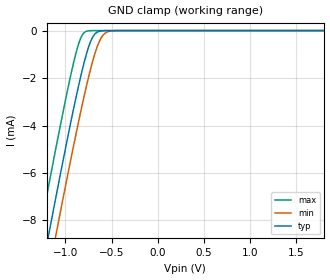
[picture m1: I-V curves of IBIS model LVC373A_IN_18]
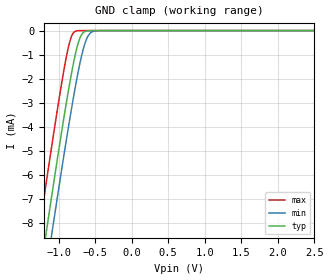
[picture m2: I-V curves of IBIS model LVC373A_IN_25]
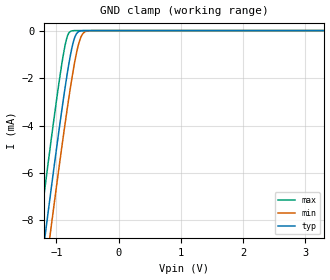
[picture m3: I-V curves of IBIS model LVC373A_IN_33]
| TEXAS INSTRUMENTS INCORPORATED
| Standard Linear and Logic Group
| IBIS Model of SN74LVC373A
| OCTAL TRANSPARENT D-TYPE LATCHES WITH 3-STATE OUTPUTS
| This file contains package information for the following:
|  TSSOP 20-pin (PW) package as [Component] LVC373A_PW
|  SSOP 20-pin (DB) package as [Component] LVC373A_DB
|  SOIC 20-pin (DW) package as [Component] LVC373A_DW
| This device can be powered at the following Vccs:
|  1.8 volt Vcc
|  2.5 volt Vcc
|  3.3 volt Vcc
| This file provides unique models under the [Model Selector] for each Vcc.
| For operation at a specific Vcc, select the appropriate model after each
| [Model Selector] keyword.
[IBIS Ver]   3.2
[Comment char]  |_char
[File Name]   sn74lvc373a.ibs
[File Rev]   1.1 | e-die
[Date]   March 5, 2002
[Source]   Data created from TI-SPICE simulations at TI-SLL.
[Notes]   The following is an IBIS list for the LVC373A.
   Please contact sllibis@ti.com with questions and
   comments concerning SLL IBIS models.
   -As there is no power clamp diode in the Input and I/O Models,
   we removed the Pwr Clamp table data from those Models.
   -Due to the fact that the Device is 5-V Input/Output
   tolarent, the output model has some Non-Monotonic Warnings.
   - C_comp values are taken at a different test condition than
   the data sheet.
[Disclaimer] Property of Texas Instruments Incorporated.  Unauthorized
   reproduction and/or distribution is strictly prohibited.
   This product is protected under copyright law.
   Created  2002, (C) Copyright  2002, Texas Instruments
   Incorporated, All Rights Reserved
   UNLESS THERE IS A SIGNED, WRITTEN AGREEMENT TO THE
   CONTRARY, TEXAS INSTRUMENTS (TI) IS PROVIDING THE IBIS
   MODELS  AND WITHOUT ANY WARRANTY, EXPRESSED OR
   IMPLIED.  TI assumes no liability for:
   1) the accuracy of the IBIS models provided to your
   company;
   2) the proper functioning of these IBIS Models in your
   design or for any resulting applications; or
   3) infringement of patents, copyrights or intellectual
   property rights resulting from your use of these IBIS
   models.
   TI provides IBIS Models as a service to our customers.
   You and your company shall not distribute, sell or give
   these models to anyone else without prior written
   permission from TI.
   TI reserves the right to make changes to our products or
   to discontinue any semiconductor product or service
   without notice, and advises our customers to obtain the
   latest version of relevant information to verify, before
   placing orders, that the information being relied on is
   current.
   Please be aware that your receipt and use of the IBIS
   information provided shall serve as acceptance of these
   terms and conditions.  If you do not accept these terms,
   you should return or destroy the IBIS models and any
   other accompanying information immediately.
| Component LVC373A_PW 20-pin TSSOP
[Component]   LVC373A_PW
[Manufacturer]   Texas Instruments, Inc.
[Package]
|   typ   min   max
R_pkg   4.500e-02   3.600e-02   5.700e-02
L_pkg   2.694e-09   2.290e-09   3.177e-09
C_pkg   1.560e-13   7.600e-14   2.590e-13
[Pin]   signal_name   model_name   R_pin   L_pin   C_pin
1   NOE   LVC373A_CTL   3.600e-02   3.045e-09   2.590e-13
2   1Q   LVC373A_OUT   5.100e-02   3.013e-09   1.890e-13
3   1D   LVC373A_IN   4.400e-02   2.695e-09   1.640e-13
4   2D   LVC373A_IN   4.700e-02   2.362e-09   7.900e-14
5   2Q   LVC373A_OUT   4.700e-02   2.333e-09   8.600e-14
6   3Q   LVC373A_OUT   4.700e-02   2.298e-09   8.500e-14
7   3D   LVC373A_IN   4.700e-02   2.351e-09   7.900e-14
8   4D   LVC373A_IN   4.400e-02   2.706e-09   1.650e-13
9   4Q   LVC373A_OUT   4.900e-02   2.999e-09   1.880e-13
10   GND   GND   3.900e-02   3.039e-09   2.570e-13
11   LE   LVC373A_CTL   3.800e-02   3.044e-09   2.580e-13
12   5Q   LVC373A_OUT   5.700e-02   3.177e-09   1.990e-13
13   5D   LVC373A_IN   4.400e-02   2.825e-09   1.730e-13
14   6D   LVC373A_IN   4.700e-02   2.429e-09   8.300e-14
15   6Q   LVC373A_OUT   4.900e-02   2.383e-09   9.000e-14
16   7Q   LVC373A_OUT   4.900e-02   2.347e-09   8.900e-14
17   7D   LVC373A_IN   4.700e-02   2.290e-09   7.600e-14
18   8D   LVC373A_IN   4.500e-02   2.613e-09   1.580e-13
19   8Q   LVC373A_OUT   4.400e-02   2.883e-09   1.810e-13
20   VCC   POWER   3.900e-02   3.044e-09   2.560e-13
| Component LVC373A_DB 20-pin SSOP
[Component]   LVC373A_DB
[Manufacturer]   Texas Instruments, Inc.
[Package]
|   typ   min   max
R_pkg   4.000e-02   3.500e-02   5.100e-02
L_pkg   3.495e-09   3.035e-09   4.314e-09
C_pkg   4.200e-13   3.460e-13   5.020e-13
[Pin]   signal_name   model_name   R_pin   L_pin   C_pin
1   NOE   LVC373A_CTL   4.900e-02   4.310e-09   5.020e-13
2   1Q   LVC373A_OUT   4.800e-02   3.903e-09   4.870e-13
3   1D   LVC373A_IN   3.500e-02   3.189e-09   3.960e-13
4   2D   LVC373A_IN   3.500e-02   3.036e-09   3.470e-13
5   2Q   LVC373A_OUT   3.500e-02   3.035e-09   3.670e-13
6   3Q   LVC373A_OUT   3.500e-02   3.035e-09   3.670e-13
7   3D   LVC373A_IN   3.500e-02   3.036e-09   3.470e-13
8   4D   LVC373A_IN   3.500e-02   3.189e-09   3.970e-13
9   4Q   LVC373A_OUT   4.700e-02   3.899e-09   4.880e-13
10   GND   GND   5.100e-02   4.314e-09   5.000e-13
11   LE   LVC373A_CTL   5.100e-02   4.314e-09   5.000e-13
12   5Q   LVC373A_OUT   4.700e-02   3.899e-09   4.880e-13
13   5D   LVC373A_IN   3.500e-02   3.189e-09   3.970e-13
14   6D   LVC373A_IN   3.500e-02   3.036e-09   3.460e-13
15   6Q   LVC373A_OUT   3.500e-02   3.035e-09   3.670e-13
16   7Q   LVC373A_OUT   3.500e-02   3.035e-09   3.670e-13
17   7D   LVC373A_IN   3.500e-02   3.036e-09   3.460e-13
18   8D   LVC373A_IN   3.500e-02   3.189e-09   3.970e-13
19   8Q   LVC373A_OUT   4.700e-02   3.899e-09   4.880e-13
20   VCC   POWER   5.100e-02   4.314e-09   5.020e-13
| Component LVC373A_DW 20-pin SOIC
[Component]   LVC373A_DW
[Manufacturer]   Texas Instruments, Inc.
[Package]
|   typ   min   max
R_pkg   3.800e-02   3.300e-02   4.500e-02
L_pkg   5.012e-09   4.110e-09   6.349e-09
C_pkg   7.170e-13   5.300e-13   8.680e-13
[Pin]   signal_name   model_name   R_pin   L_pin   C_pin
1   NOE   LVC373A_CTL   4.200e-02   6.336e-09   8.650e-13
2   1Q   LVC373A_OUT   4.300e-02   5.542e-09   8.670e-13
3   1D   LVC373A_IN   3.400e-02   4.714e-09   7.320e-13
4   2D   LVC373A_IN   3.400e-02   4.377e-09   5.910e-13
5   2Q   LVC373A_OUT   3.600e-02   4.130e-09   5.330e-13
6   3Q   LVC373A_OUT   3.500e-02   4.111e-09   5.300e-13
7   3D   LVC373A_IN   3.400e-02   4.284e-09   5.830e-13
8   4D   LVC373A_IN   3.400e-02   4.634e-09   7.260e-13
9   4Q   LVC373A_OUT   4.000e-02   5.518e-09   8.650e-13
10   GND   GND   4.300e-02   6.349e-09   8.660e-13
11   LE   LVC373A_CTL   4.100e-02   6.281e-09   8.610e-13
12   5Q   LVC373A_OUT   4.500e-02   5.561e-09   8.680e-13
13   5D   LVC373A_IN   3.300e-02   4.778e-09   7.420e-13
14   6D   LVC373A_IN   3.500e-02   4.414e-09   5.960e-13
15   6Q   LVC373A_OUT   3.500e-02   4.110e-09   5.330e-13
16   7Q   LVC373A_OUT   3.600e-02   4.130e-09   5.330e-13
17   7D   LVC373A_IN   3.400e-02   4.377e-09   5.910e-13
18   8D   LVC373A_IN   3.400e-02   4.714e-09   7.310e-13
19   8Q   LVC373A_OUT   4.300e-02   5.569e-09   8.680e-13
20   VCC   POWER   4.200e-02   6.308e-09   8.640e-13
| Model LVC373A_IN
[Model Selector]   LVC373A_IN
LVC373A_IN_18   1.8 volt Vcc
LVC373A_IN_25   2.5 volt Vcc
LVC373A_IN_33   3.3 volt Vcc
| Model LVC373A_CTL
[Model Selector]   LVC373A_CTL
LVC373A_CTL_18   1.8 volt Vcc
LVC373A_CTL_25   2.5 volt Vcc
LVC373A_CTL_33   3.3 volt Vcc
| Model LVC373A_OUT
[Model Selector]   LVC373A_OUT
LVC373A_OUT_18   1.8 volt Vcc
LVC373A_OUT_25   2.5 volt Vcc
LVC373A_OUT_33   3.3 volt Vcc
| Models and submodels in the file (9): LVC373A_IN_18 (Input), LVC373A_IN_25 (Input), LVC373A_IN_33 (Input), LVC373A_CTL_18 (Input), LVC373A_CTL_25 (Input), LVC373A_CTL_33 (Input), LVC373A_OUT_18 (3-state), LVC373A_OUT_25 (3-state), LVC373A_OUT_33 (3-state)
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[Model]   LVC373A_IN_18
Model_type  Input
Vinl=0.5775
Vinh=1.2675
| variable   typ   min   max
C_comp   6.13pF   2.27pF   8.42pF
[Temperature Range]   40   100   -40
| Ambient temperature   25   85   -40
[Voltage range]   1.8   1.65   1.95
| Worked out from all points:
|   GND clamp passes 1 mA (typ) near -0.77 V on its own axis
[GND Clamp]
| LVC373A_IN_18
|   Voltage   I(typ)   I(min)   I(max)
-5V       -90.43mA   -91.87mA   -88.61mA
-1.295V   -10.95mA   -12.54mA   -8.886mA
-1.26V    -10.22mA   -11.82mA   -8.161mA
-1.17V    -8.383mA   -9.982mA   -6.315mA
-1.095V   -6.868mA   -8.465mA   -4.803mA
-930mV    -3.652mA   -5.216mA   -1.678mA
-835mV    -1.957mA   -3.443mA   -332.7uA
-765mV    -899.4uA   -2.23mA    -22.13uA
-705mV    -284.6uA   -1.306mA   -1.254uA
-635mV    -34.23uA   -487.3uA   -41.86nA
-565mV    -2.862uA   -99.75uA   -1.396nA
1.8V      4.942pA    12.9pA     4.394pA
[Model]   LVC373A_IN_25
Model_type  Input
Vinl=0.7
Vinh=1.7
| variable   typ   min   max
C_comp   6.14pF   2.32pF   8.41pF
[Temperature Range]   40   100   -40
| Ambient temperature   25   85   -40
[Voltage range]   2.5   2.3   2.7
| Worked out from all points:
|   GND clamp passes 1 mA (typ) near -0.77 V on its own axis
[GND Clamp]
| LVC373A_IN_25
|   Voltage   I(typ)   I(min)   I(max)
-5V       -90.43mA   -91.87mA   -88.61mA
-1.265V   -10.33mA   -11.92mA   -8.265mA
-1.17V    -8.383mA   -9.982mA   -6.315mA
-1.095V   -6.868mA   -8.465mA   -4.803mA
-1.07V    -6.369mA   -7.964mA   -4.307mA
-930mV    -3.652mA   -5.216mA   -1.678mA
-830mV    -1.874mA   -3.353mA   -288.1uA
-760mV    -835.1uA   -2.148mA   -17.53uA
-705mV    -284.6uA   -1.306mA   -1.254uA
-630mV    -28.82uA   -444.4uA   -32.83nA
-555mV    -1.996uA   -76.09uA   -860.6pA
2.5V      7.019pA    15.03pA    6.445pA
[Model]   LVC373A_IN_33
Model_type  Input
Vinl=0.8
Vinh=2.0
| variable   typ   min   max
C_comp   6.15pF   2.29pF   8.40pF
[Temperature Range]   40   100   -40
| Ambient temperature   25   85   -40
[Voltage range]   3.3   3   3.6
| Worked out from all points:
|   GND clamp passes 1 mA (typ) near -0.77 V on its own axis
[GND Clamp]
| LVC373A_IN_33
|   Voltage   I(typ)   I(min)   I(max)
-5V       -90.43mA   -91.87mA   -88.61mA
-1.275V   -10.53mA   -12.13mA   -8.472mA
-1.18V    -8.586mA   -10.18mA   -6.518mA
-1.1V     -6.968mA   -8.566mA   -4.902mA
-885mV    -2.825mA   -4.363mA   -951.4uA
-825mV    -1.792mA   -3.264mA   -247.4uA
-765mV    -899.4uA   -2.23mA    -22.13uA
-700mV    -251.1uA   -1.236mA   -984.3nA
-635mV    -34.23uA   -487.3uA   -41.86nA
-585mV    -5.874uA   -166.8uA   -3.688nA
-510mV    -392.6nA   -20.95uA   -100.7pA
3.3V      9.4pA      17.51pA    8.777pA
